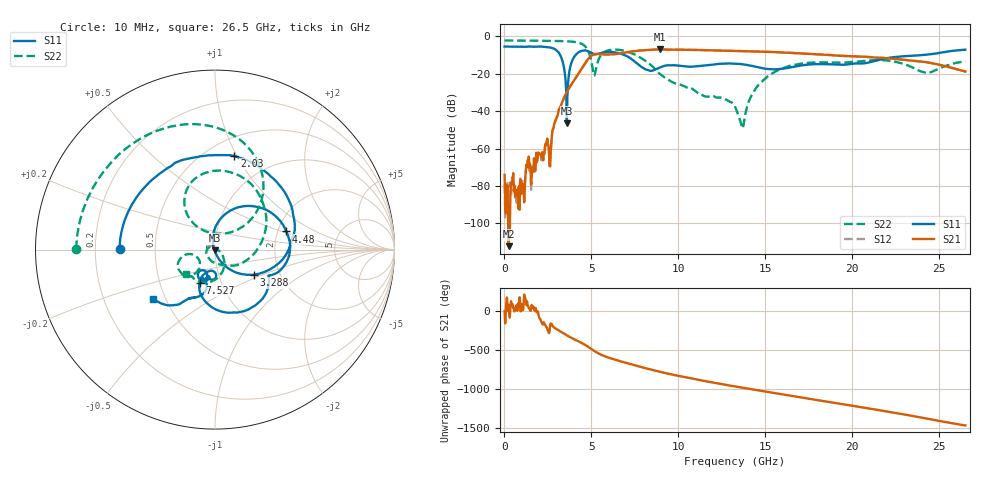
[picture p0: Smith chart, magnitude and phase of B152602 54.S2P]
!  2-Port S-parameters saved by WinCal
! VAR MeasName=S-Parameters (CALIBRATED_DATA) read from VNA (N5242A)
! VAR MeasDate=2016-1-5 16:33:45
! VAR NAME=B152602 54
! VAR FILENAME=B152602 54.S2P
! VAR DATE=2016-1-5 16:33:45
! VAR PHYS_PORTS=1,2
# Hz S DB R 50
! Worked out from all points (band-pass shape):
!   801 points, 10 MHz to 26.5 GHz, reference 50 ohm
!   highest |S21| = -7.04 dB at 8.95 GHz (marker M1); lowest = -112.1 dB at 241.8 MHz (marker M2)
!   |S21| within 3 dB of the highest: 5.057 GHz to 18.76 GHz (13.7 GHz wide, 115 % of centre)
!   lowest |S11| = -46.5 dB at 3.586 GHz (marker M3), VSWR 1.01, Z = 49.7 - j0.397 ohm
!   |S11| at or under -10 dB: 3.202 GHz to 4.09 GHz (887.2 MHz wide, 24.3 % of centre); 6.892 GHz to 24.06 GHz (17.17 GHz wide, 111 % of centre)
!   |S22| runs from -49.3 to -2.2 dB; largest |S21 - S12| = 0.0033
!   S11 on the Smith chart (normalised r, x): 10 MHz: 0.31, +0.00; 2.03 GHz: 0.67, +0.98; 3.288 GHz: 1.47, -0.44; 4.48 GHz: 2.23, +0.54; 7.527 GHz: 0.79, -0.31; 26.5 GHz: 0.43, -0.29
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1e7  -5.50 179.5  -74.04 0.3  -79.23 110.2  -2.23 179.8
2.417875e8  -5.51 168.4  -112.13 77.6  -85.83 30.1  -2.25 176.2
1.0696e9  -5.63 129.3  -78.92 13.2  -78.29 58.9  -2.30 163.4
2.029862e9  -5.48 78.4  -63.08 -95.4  -62.36 -93.2  -2.39 147.7
2.625888e9  -5.99 38.1  -69.50 -176.3  -69.30 -168.2  -2.45 136.7
3.288138e9  -11.82 -33.1  -36.01 91.8  -36.04 92.0  -2.58 121.9
3.58615e9  -46.50 -122.5  -29.83 51.3  -29.83 51.3  -2.69 113.9
3.917275e9  -12.57 68.2  -24.81 10.4  -24.81 10.5  -2.90 102.9
4.447075e9  -7.81 17.1  -17.15 -48.0  -17.14 -47.9  -4.06 77.1
4.480188e9  -7.74 14.3  -16.68 -51.9  -16.66 -51.8  -4.22 74.9
5.17555e9  -9.53 -25.5  -9.58 -151.4  -9.57 -151.3  -20.95 92.2
5.904025e9  -8.36 -48.7  -9.75 131.5  -9.74 131.5  -7.69 105.1
7.526538e9  -13.76 -114.8  -7.86 24.3  -7.82 24.4  -9.89 26.6
8.851038e9  -17.06 -87.4  -7.06 -52.3  -7.04 -52.3  -19.45 -54.6
8.950375e9  -16.64 -87.4  -7.04 -57.7  -7.02 -57.8  -20.25 -61.4
1.116891e10  -15.92 -101.4  -7.35 -161.0  -7.32 -160.9  -30.54 160.8
1.3255e10  -14.65 -116.8  -7.85 115.7  -7.83 115.6  -37.60 161.4
1.368546e10  -14.97 -121.6  -7.96 99.3  -7.91 99.1  -49.25 64.7
1.500996e10  -17.33 -122.7  -8.28 49.4  -8.28 49.1  -22.43 -48.9
1.769208e10  -14.95 -110.2  -9.49 -49.2  -9.46 -49.0  -14.08 -113.7
2.209604e10  -11.51 -106.6  -11.83 150.1  -11.77 150.0  -13.02 -157.7
2.65e10  -7.14 -141.7  -18.85 -24.9  -18.83 -25.2  -13.45 -140.0
